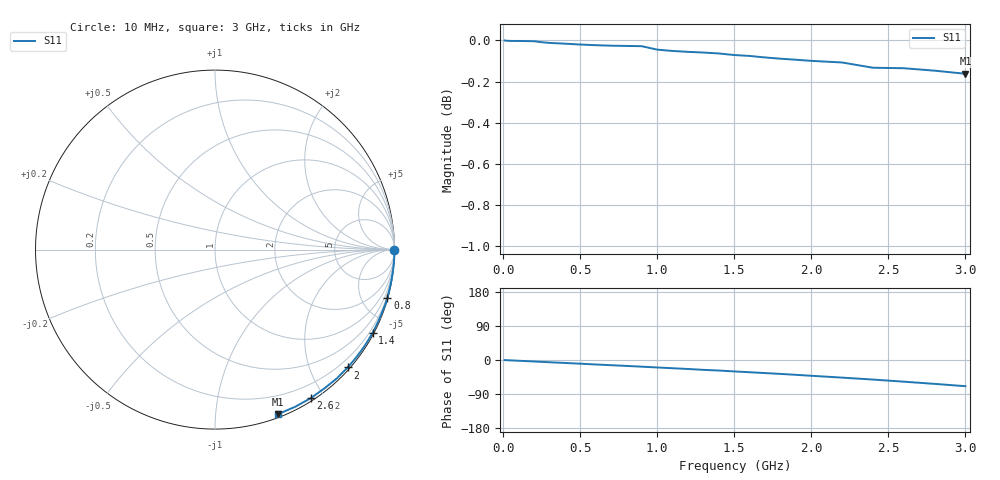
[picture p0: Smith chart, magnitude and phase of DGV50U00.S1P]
! SIEMENS Small Signal Semiconductors
! BAV70
! Silicon Switching Diode in SOT23
! VR = 0.5 V
! S-Parameters:  May  1995
# GHz  S  MA  R  50
!  f  S11
! GHz  MAG  ANG
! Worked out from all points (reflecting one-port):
!   30 points, 10 MHz to 3 GHz, reference 50 ohm
!   lowest |S11| = -0.2 dB at 3 GHz (marker M1), VSWR 107.17, Z = 1.45 - j72.6 ohm
!   phase of S11 starts at -0 deg and turns -69 deg over the sweep
!   S11 on the Smith chart (normalised r, x): 10 MHz: open; 800 MHz: 0.08, -7.30; 1.4 GHz: 0.06, -4.04; 2 GHz: 0.05, -2.63; 2.6 GHz: 0.03, -1.83; 3 GHz: 0.03, -1.45
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0.01  1 -0.2
0.1  0.9997 -2.0
0.15  0.9996 -2.9
0.2  0.9996 -3.9
0.25  0.999 -4.9
0.3  0.9986 -5.9
0.4  0.9982 -7.8
0.5  0.9977 -9.7
0.6  0.9973 -11.8
0.7  0.9971 -13.7
0.8  0.9969 -15.6
0.9  0.9968 -17.6
1  0.9949 -19.7
1.1  0.9941 -21.7
1.2  0.9936 -23.7
1.3  0.9932 -26.0
1.4  0.9927 -27.8
1.5  0.9919 -30.1
1.6  0.9914 -32.3
1.7  0.9905 -34.5
1.8  0.9898 -36.7
1.9  0.9893 -39.1
2  0.9886 -41.6
2.2  0.9877 -46.5
2.4  0.9848 -51.6
2.6  0.9846 -57.2
2.8  0.9832 -63.0
3  0.9815 -69.1
